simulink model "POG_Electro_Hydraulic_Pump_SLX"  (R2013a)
settings: Solver=ode45  StartTime=0.0  StopTime=10.0  MaxStep=0.001  RelTol=1e-3
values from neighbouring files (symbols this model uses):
  b_m = 0.02*Nm/(100*rpm)    [POG_Electro_Hydraulic_Pump_NL_SLX_m.m]    (also in POG_Electro_Hydraulic_Pump_Rele_SLX_m.m; POG_Electro_Hydraulic_Pump_SLX_m.m = 1)
  d_0 = (4*mm)^3/sec/(10*atm)    [POG_Electro_Hydraulic_Pump_NL_SLX_m.m]    (also in POG_Electro_Hydraulic_Pump_Rele_SLX_m.m; POG_Electro_Hydraulic_Pump_SLX_m.m = 1)
  F_2_0 = 0    [POG_Electro_Hydraulic_Pump_NL_SLX_m.m]    (also in POG_Electro_Hydraulic_Pump_Rele_SLX_m.m; POG_Electro_Hydraulic_Pump_SLX_m.m)
  J_m = 1*cm^2*1*kg    [POG_Electro_Hydraulic_Pump_NL_SLX_m.m]    (also in POG_Electro_Hydraulic_Pump_Rele_SLX_m.m; POG_Electro_Hydraulic_Pump_SLX_m.m = 1)
  K_0 = 100*atm/((10*cm)^3)    [POG_Electro_Hydraulic_Pump_NL_SLX_m.m]    (also in POG_Electro_Hydraulic_Pump_Rele_SLX_m.m; POG_Electro_Hydraulic_Pump_SLX_m.m = 1)
  K_m = 0.5    [POG_Electro_Hydraulic_Pump_NL_SLX_m.m]    (also in POG_Electro_Hydraulic_Pump_Rele_SLX_m.m; POG_Electro_Hydraulic_Pump_SLX_m.m = 1; POG_Hydraulic_Clutch_NL_2_SLX_m.m = 16887.5; POG_Hydraulic_Clutch_SS_NL_SLX_m.m = P_a_0*A/(3*cm))
  K_p = 5e-06    [POG_Electro_Hydraulic_Pump_NL_SLX_m.m]    (also in POG_Electro_Hydraulic_Pump_Rele_SLX_m.m; POG_Electro_Hydraulic_Pump_SLX_m.m = 1)
  L_a = 0.3*mHenry    [POG_Electro_Hydraulic_Pump_NL_SLX_m.m]    (also in POG_Electro_Hydraulic_Pump_Rele_SLX_m.m; POG_Electro_Hydraulic_Pump_SLX_m.m = 1)
  P_6_0 = 0    [POG_Electro_Hydraulic_Pump_NL_SLX_m.m]    (also in POG_Electro_Hydraulic_Pump_Rele_SLX_m.m; POG_Electro_Hydraulic_Pump_SLX_m.m; POG_Hydraulic_Clutch_SS_NL_SLX_m.m; POG_Hydraulic_Clutch_SS_SLX_m.m)
  Q_b_0 = 0    [POG_Electro_Hydraulic_Pump_SLX_m.m]
  R_a = 1*Ohm    [POG_Electro_Hydraulic_Pump_NL_SLX_m.m]    (also in POG_Electro_Hydraulic_Pump_Rele_SLX_m.m; POG_Electro_Hydraulic_Pump_SLX_m.m = 1)
  Ts = Tfin/Nr_Ts_Points    (= 0.03)    [POG_Electro_Hydraulic_Pump_NL_SLX_m.m]    (also in POG_Electro_Hydraulic_Pump_Rele_SLX_m.m = 0.035; POG_Electro_Hydraulic_Pump_SLX_m.m = 0.005; POG_Hydraulic_Clutch_NL_2_SLX_m.m = 0.0002; POG_Hydraulic_Clutch_SS_NL_SLX_m.m = 0.0002)
  V_0_0 = 0    [POG_Electro_Hydraulic_Pump_SLX_m.m]
  V_1_0_0 = 0    [POG_Electro_Hydraulic_Pump_NL_SLX_m.m]    (also in POG_Electro_Hydraulic_Pump_Rele_SLX_m.m; POG_Electro_Hydraulic_Pump_SLX_m.m)

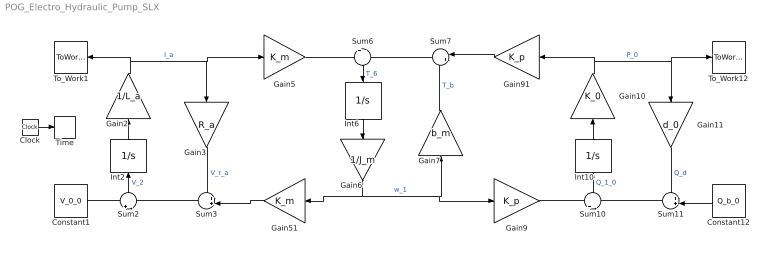
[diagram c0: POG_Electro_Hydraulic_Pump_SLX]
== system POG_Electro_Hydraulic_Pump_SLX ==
  Clock : Clock
  Constant1 : Constant  Value=V_0_0
  Constant12 : Constant  Value=Q_b_0
  Gain10 : Gain  Gain=K_0  Multiplication=Matrix(K*u)
  Gain11 : Gain  Gain=d_0  Multiplication=Matrix(K*u)
  Gain2 : Gain  Gain=1/L_a  Multiplication=Matrix(K*u)
  Gain3 : Gain  Gain=R_a  Multiplication=Matrix(K*u)
  Gain5 : Gain  Gain=K_m  Multiplication=Matrix(K*u)
  Gain51 : Gain  Gain=K_m  Multiplication=Matrix(K*u)
  Gain6 : Gain  Gain=1/J_m  Multiplication=Matrix(K*u)
  Gain7 : Gain  Gain=b_m  Multiplication=Matrix(K*u)
  Gain9 : Gain  Gain=K_p  Multiplication=Matrix(K*u)
  Gain91 : Gain  Gain=K_p  Multiplication=Matrix(K*u)
  Int10 : Integrator  InitialCondition=V_1_0_0
  Int2 : Integrator  InitialCondition=F_2_0
  Int6 : Integrator  InitialCondition=P_6_0
  Sum10 : Sum  Inputs=+|-
  Sum11 : Sum  Inputs=++|
  Sum2 : Sum  Inputs=+|-
  Sum3 : Sum  Inputs=++|
  Sum6 : Sum  Inputs=+|-
  Sum7 : Sum  Inputs=|++
  Time : ToWorkspace  VariableName=t  SampleTime=Ts
  To_Work1 : ToWorkspace  VariableName=I_0_0  SampleTime=Ts
  To_Work12 : ToWorkspace  VariableName=P_b_0  SampleTime=Ts
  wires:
  Constant1/1 -> Sum2/1
  Sum3/1 -> Sum2/2
  Gain2/1 -> To_Work1/1, Gain3/1, Gain5/1  "I_a"
  Sum2/1 -> Int2/1  "V_2"
  Int2/1 -> Gain2/1
  Gain51/1 -> Sum3/2
  Gain3/1 -> Sum3/1  "V_r_a"
  Gain5/1 -> Sum6/1
  Gain6/1 -> Gain51/1, Gain7/1, Gain9/1  "w_1"
  Sum7/1 -> Sum6/2
  Sum6/1 -> Int6/1  "T_6"
  Int6/1 -> Gain6/1
  Gain91/1 -> Sum7/1
  Gain7/1 -> Sum7/2  "T_b"
  Gain9/1 -> Sum10/1
  Gain10/1 -> Gain91/1, To_Work12/1, Gain11/1  "P_0"
  Sum11/1 -> Sum10/2
  Sum10/1 -> Int10/1  "Q_1_0"
  Int10/1 -> Gain10/1
  Constant12/1 -> Sum11/2
  Gain11/1 -> Sum11/1  "Q_d"
  Clock/1 -> Time/1
